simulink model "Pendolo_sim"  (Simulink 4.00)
settings: Solver=ode45  StartTime=0.0  StopTime=Tf  RelTol=1e-3
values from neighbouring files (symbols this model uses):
  csi = 0.05    [pendolo.m]    (also in pendolo_param.m)
  g = 9.81    [pendolo.m]    (also in pendolo_param.m)
  L = 1    [pendolo.m]    (also in pendolo_param.m)
  lambda = 1.3    [pendolo.m]    (also in pendolo_param.m)
  r = 1.4    [pendolo.m]    (also in pendolo_param.m)
  x0 = 0    [pendolo.m]    (also in pendolo_param.m)
  xp0 = 0    [pendolo.m]    (also in pendolo_param.m)

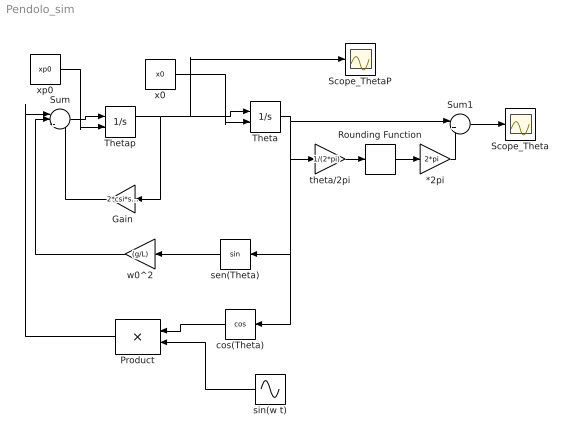
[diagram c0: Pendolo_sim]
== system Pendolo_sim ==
  *2pi : Gain  Gain=2*pi  Multiplication=Element-wise(K.*u)  SaturateOnIntegerOverflow=on
  Gain : Gain  Orientation=left  Gain=2*csi*sqrt(g/L)  Multiplication=Element-wise(K.*u)  SaturateOnIntegerOverflow=on
  Product : Product  Orientation=left  Inputs=2  Multiplication=Element-wise(.*)  SaturateOnIntegerOverflow=on
  Rounding Function : Rounding  Operator=round
  Scope_Theta : Scope
  Scope_ThetaP : Scope
  Sum : Sum  Inputs=|+--  SaturateOnIntegerOverflow=on
  Sum1 : Sum  Inputs=|+-  SaturateOnIntegerOverflow=on
  Theta : Integrator  ExternalReset=none  InitialConditionSource=external  InitialCondition=0  LimitOutput=off  UpperSaturationLimit=inf  LowerSaturationLimit=-inf  ShowSaturationPort=off  ShowStatePort=off  AbsoluteTolerance=auto
  Thetap : Integrator  ExternalReset=none  InitialConditionSource=external  InitialCondition=0  LimitOutput=off  UpperSaturationLimit=inf  LowerSaturationLimit=-inf  ShowSaturationPort=off  ShowStatePort=off  AbsoluteTolerance=auto
  cos(Theta) : Trigonometry  Orientation=left  Operator=cos  OutputSignalType=auto
  sen(Theta) : Trigonometry  Orientation=left  Operator=sin  OutputSignalType=auto
  sin(w t) : Sin  Orientation=left  SineType=Time-based  Amplitude=(r*sqrt(g/L))^2*lambda  Bias=0  Frequency=r*sqrt(g/L)  Phase=0  Samples=10  SampleTime=0
  theta/2pi : Gain  Gain=1/(2*pi)  Multiplication=Element-wise(K.*u)  SaturateOnIntegerOverflow=on
  w0^2 : Gain  Orientation=left  Gain=(g/L)  Multiplication=Element-wise(K.*u)  SaturateOnIntegerOverflow=on
  x0 : Constant  Value=x0
  xp0 : Constant  Value=xp0
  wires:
  Thetap/1 -> Gain/1, Theta/1, Scope_ThetaP/1
  Sum/1 -> Thetap/1
  Gain/1 -> Sum/3
  Theta/1 -> sen(Theta)/1, cos(Theta)/1, theta/2pi/1, Sum1/1
  sen(Theta)/1 -> w0^2/1
  w0^2/1 -> Sum/2
  cos(Theta)/1 -> Product/1
  sin(w t)/1 -> Product/2
  Product/1 -> Sum/1
  xp0/1 -> Thetap/2
  x0/1 -> Theta/2
  theta/2pi/1 -> Rounding Function/1
  Sum1/1 -> Scope_Theta/1
  Rounding Function/1 -> *2pi/1
  *2pi/1 -> Sum1/2
